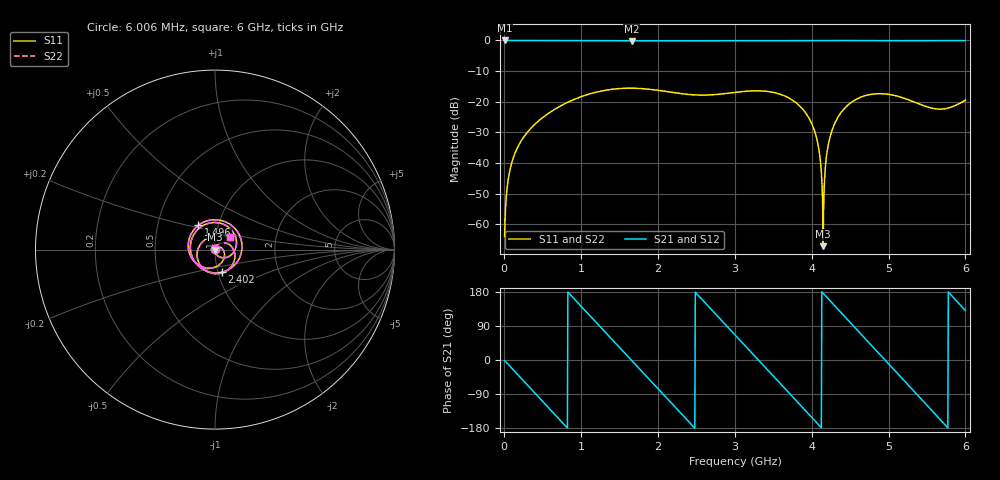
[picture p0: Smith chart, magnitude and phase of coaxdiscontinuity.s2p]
! TOUCHSTONE file generated by CST MICROWAVE STUDIO
! Date and time: Tue Dec 30 06:16:18 2014
! Project name: coaxdiscontinuity.cst
! Port labels:
! Port 1 = ""
! Port 2 = ""
# GHZ S MA R 50
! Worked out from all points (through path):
!   999 points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, 6.006 MHz to 6 GHz, reference 50 ohm
!   highest |S21| = 0.00 dB at 6.006 MHz (marker M1); lowest = -0.1 dB at 1.658 GHz (marker M2)
!   group delay of S21, straight-line fit = 606 ps
!   lowest |S11| = -67.1 dB at 4.15 GHz (marker M3), VSWR 1.00, Z = 50 + j0.00617 ohm
!   |S11| at or under -10 dB: start of sweep to end of sweep
!   |S22| runs from -67.2 to -15.6 dB; largest |S21 - S12| = 0
!   S11 on the Smith chart (normalised r, x): 6.006 MHz: 1.00, +0.00; 1.496 GHz: 0.80, +0.22; 2.402 GHz: 1.05, -0.27; 6 GHz: 1.16, +0.16
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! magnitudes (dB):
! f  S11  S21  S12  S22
! 6.006 MHz  -64.0  0.0  0.0  -64.0
! 42.04 MHz  -47.3  0.0  0.0  -47.3
! 72.07 MHz  -42.6  0.0  0.0  -42.6
! 222.2 MHz  -32.7  0.0  0.0  -32.7
! 534.5 MHz  -24.5  0.0  0.0  -24.5
! 1.009 GHz  -18.3  -0.1  -0.1  -18.3
! 1.496 GHz  -15.7  -0.1  -0.1  -15.7
! 1.658 GHz  -15.6  -0.1  -0.1  -15.6
! 2.006 GHz  -16.3  -0.1  -0.1  -16.3
! 2.402 GHz  -17.6  -0.1  -0.1  -17.6
! 3.009 GHz  -16.9  -0.1  -0.1  -16.9
! 3.646 GHz  -18.1  -0.1  -0.1  -18.1
! 4.006 GHz  -27.4  0.0  0.0  -27.4
! 4.09 GHz  -34.9  0.0  0.0  -34.9
! 4.132 GHz  -45.4  0.0  0.0  -45.4
! 4.15 GHz  -67.1  0.0  0.0  -67.2
! 4.222 GHz  -33.3  0.0  0.0  -33.3
! 4.36 GHz  -24.3  0.0  0.0  -24.3
! 4.631 GHz  -18.6  -0.1  -0.1  -18.6
! 5.003 GHz  -17.6  -0.1  -0.1  -17.6
! 5.634 GHz  -22.4  0.0  0.0  -22.4
! 6 GHz  -19.5  0.0  0.0  -19.5
